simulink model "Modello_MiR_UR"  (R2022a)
settings: Solver=FixedStepAuto  StartTime=0.0  StopTime=time_s(end,1)  FixedStep=Sim.dt*10  RelTol=1e-3  EnableMultiTasking=on
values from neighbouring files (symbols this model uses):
  a = 0.250    (= 0.25)    [Modello_MiR_UR_script.m]    (also in Modello_MiR_2ruote_script.m; Modello_MiR_6ruote_script.m; Modello_MiR_6ruote_validato_script.m)
  a1 = 0.18265    [Modello_MiR_UR_script.m]    (also in UR_DHtable_e.m = 0; Modello_MiR_2ruote_script.m = deg2rad(5); Modello_MiR_6ruote_script.m = deg2rad(5); Modello_MiR_6ruote_validato_script.m)
  a2 = 0.40857    [Modello_MiR_UR_script.m]    (also in UR_DHtable_e.m = 612; Modello_MiR_2ruote_script.m = deg2rad(25); Modello_MiR_6ruote_script.m = deg2rad(25); Modello_MiR_6ruote_validato_script.m)
  Att_C1 = 0.01    [Modello_MiR_UR_script.m]    (also in Modello_MiR_6ruote_validato_script.m)
  Att_C2 = 0.01    [Modello_MiR_UR_script.m]    (also in Modello_MiR_6ruote_validato_script.m)
  Att_C5 = 0.01    [Modello_MiR_UR_script.m]    (also in Modello_MiR_6ruote_validato_script.m)
  Att_C6 = 0.01    [Modello_MiR_UR_script.m]    (also in Modello_MiR_6ruote_validato_script.m)
  b = 0.1875    [Modello_MiR_UR_script.m]    (also in Modello_MiR_2ruote_script.m; Modello_MiR_6ruote_script.m; Modello_MiR_6ruote_validato_script.m)
  b_caster = 0.07    [Modello_MiR_UR_script.m]    (also in Modello_MiR_2ruote_script.m; Modello_MiR_6ruote_script.m; Modello_MiR_6ruote_validato_script.m)
  bd = 0.205    [Modello_MiR_UR_script.m]    (also in Modello_MiR_2ruote_script.m; Modello_MiR_6ruote_script.m; Modello_MiR_6ruote_validato_script.m)
  F23MIR = @(u) (mv*9.801/4)-(mv*h*u(5)+(mv*9.801/4)*(2*a-b_caster*(cos(u(1))+cos(u(2)))))/(4*a-b_caster*(cos(u(1))+cos(u(2)))+b_caster*(cos(u(3))+cos(u(4))))    [Modello_MiR_UR_script.m]
  F23UR5 = @(u) (u(7)/4)-u(11)    [Modello_MiR_UR_script.m]
  F43MIR = @(u) (1/(2*bd))*(mv*u(6)*h+((mv*h*u(5)+(mv*9.801/4)*(2*a-b_caster*(cos(u(1))+cos(u(2)))))/(4*a-b_caster*(cos(u(1))+cos(u(2)))+b_caster*(cos(u(3))+cos(u(4)))))*(2*bd-b_caster*(sin(u(3))+sin(u(4))))+((mv*9.801/4)-(mv*h*u(5)+(mv*9.801/4)*(2*a-b_caster*(cos(u(1))+cos(u(2)))))/(4*a-b_caster*(cos(u(1))+cos(u(2)))+b_caster*(cos(u(3))+cos(u(4)))))*(2*bd-b_caster*(sin(u(1))+sin(u(2)))))    [Modello_MiR_UR_script.m]
  F43UR5 = @(u) (1/(2*bd))*(u(8) - u(6)*H +u(11)*(2*bd-b_caster*(sin(u(3))+sin(u(4))))+u(12)*(2*bd-b_caster*(sin(u(1))+sin(u(2)))))    [Modello_MiR_UR_script.m]
  F63MIR = @(u) (mv*h*u(5)+(mv*9.801/4)*(2*a-b_caster*(cos(u(1))+cos(u(2)))))/(4*a-b_caster*(cos(u(1))+cos(u(2)))+b_caster*(cos(u(3))+cos(u(4))))    [Modello_MiR_UR_script.m]
  F63UR5 = @(u)(-a*u(7)/2 -u(5)*H -u(9) +(u(7)/4)*(2*a-b_caster*(cos(u(1))+cos(u(2)))))/(4*a-b_caster*(cos(u(1))+cos(u(2)))+b_caster*(cos(u(3))+cos(u(4))))    [Modello_MiR_UR_script.m]
  f_c = 0.29564    [Modello_MiR_UR_script.m]    (also in Modello_MiR_6ruote_validato_script.m)
  f_d3 = 0.35846    [Modello_MiR_UR_script.m]    (also in Modello_MiR_6ruote_validato_script.m)
  f_d4 = 0.2333    [Modello_MiR_UR_script.m]    (also in Modello_MiR_6ruote_validato_script.m)
  fa_c = 0.27474    [Modello_MiR_UR_script.m]    (also in Modello_MiR_6ruote_validato_script.m)
  fa_d3 = 0.3694    [Modello_MiR_UR_script.m]    (also in Modello_MiR_6ruote_validato_script.m)
  fa_d4 = 0.28065    [Modello_MiR_UR_script.m]    (also in Modello_MiR_6ruote_validato_script.m)
  fm_fun = @(u) (u <= -am2 || u >= am2) * 0 + (u > -am2 && u <= -am1) * (- u* Mza/(am2 -am1) - Mza* am2/(am2 -am1)) +           + (u > -am1 && u <= am1) * (Mza * u / am1) + (u > am1 && u < am2) * (Mza * u /(am1 -am2) - Mza * am2 /(am1 - am2))    [Modello_MiR_UR_script.m]    (also in Modello_MiR_6ruote_script.m = @(u) (u <= -am2 | u >= am2)*0 + (u > -am2 && u <= -am1)*(- u; Modello_MiR_6ruote_validato_script.m)
  Hi = 1    [UR5e_data.m]
  Icw_1 = 1/2 * mcw * rc^2    (= 0.002004225735)    [Modello_MiR_UR_script.m]    (also in Modello_MiR_2ruote_script.m; Modello_MiR_6ruote_script.m; Modello_MiR_6ruote_validato_script.m)
  Icw_2 = 1/12 * mcw * ec^2 + 1/4 * mcw * rc^2    (= 0.00104098243873)    [Modello_MiR_UR_script.m]    (also in Modello_MiR_2ruote_script.m; Modello_MiR_6ruote_script.m; Modello_MiR_6ruote_validato_script.m)
  Idw_1 = 1/2 * mdw * rd^2    (= 0.00551836278784)    [Modello_MiR_UR_script.m]    (also in Modello_MiR_2ruote_script.m; Transfer_Function_Gol_Gcl.m = Inertia_vect(jj,1); Modello_MiR_6ruote_script.m; Modello_MiR_6ruote_validato_script.m)
  iMax = 20.7*1.1    (= 22.77)    [Modello_MiR_UR_script.m]    (also in Modello_MiR_2ruote_script.m; Modello_MiR_6ruote_script.m; Modello_MiR_6ruote_validato_script.m)
  Iv = mv * (l^2 + w^2)  / 12    (= 6.75343333333)    [Modello_MiR_UR_script.m]    (also in Modello_MiR_2ruote_script.m; Modello_MiR_6ruote_script.m; Modello_MiR_6ruote_validato_script.m = 8.95033333333)
  Kc = 0.15    [Modello_MiR_UR_script.m]    (also in Modello_MiR_2ruote_script.m; Modello_MiR_6ruote_script.m; Modello_MiR_6ruote_validato_script.m)
  Ki_i = 1    [Modello_MiR_UR_script.m]    (also in Modello_MiR_2ruote_script.m; Modello_MiR_6ruote_script.m; Modello_MiR_6ruote_validato_script.m)
  Ki_v = 1    [Modello_MiR_UR_script.m]    (also in Modello_MiR_2ruote_script.m; Modello_MiR_6ruote_script.m; Modello_MiR_6ruote_validato_script.m)
  kk = 0.00005    (= 5e-05)    [Modello_MiR_UR_script.m]    (also in Modello_MiR_2ruote_script.m; Modello_MiR_6ruote_script.m; Modello_MiR_6ruote_validato_script.m)
  Kp_i = 5    [Modello_MiR_UR_script.m]    (also in Modello_MiR_2ruote_script.m; Modello_MiR_6ruote_script.m; Modello_MiR_6ruote_validato_script.m)
  Kp_v = 5    [Modello_MiR_UR_script.m]    (also in Modello_MiR_2ruote_script.m; Modello_MiR_6ruote_script.m; Modello_MiR_6ruote_validato_script.m)
  kv = 1.5e-6    (= 1.5e-06)    [Modello_MiR_UR_script.m]    (also in Modello_MiR_2ruote_script.m; Modello_MiR_6ruote_script.m; Modello_MiR_6ruote_validato_script.m)
  L = R * tauE    (= 0.00181134822805)    [Modello_MiR_UR_script.m]    (also in Modello_MiR_2ruote_script.m; Modello_MiR_6ruote_script.m; Modello_MiR_6ruote_validato_script.m)
  mcw = rc^2 * pi * ec * rhopoliu + 1    (= 1.02616357632)    [Modello_MiR_UR_script.m]    (also in Modello_MiR_2ruote_script.m; Modello_MiR_6ruote_script.m; Modello_MiR_6ruote_validato_script.m)
  mv = 83    [Modello_MiR_UR_script.m]    (also in Modello_MiR_2ruote_script.m; Modello_MiR_6ruote_script.m; Modello_MiR_6ruote_validato_script.m = 110)
  Phi1_start = psi_mir(1,1)    [Modello_MiR_UR_script.m]    (also in Modello_MiR_6ruote_validato_script.m)
  Phi2_start = psi_mir(1,1)    [Modello_MiR_UR_script.m]    (also in Modello_MiR_6ruote_validato_script.m)
  Phi5_start = psi_mir(1,1)    [Modello_MiR_UR_script.m]    (also in Modello_MiR_6ruote_validato_script.m)
  Phi6_start = psi_mir(1,1)    [Modello_MiR_UR_script.m]    (also in Modello_MiR_6ruote_validato_script.m)
  Psi_start = psi_mir(1,1)    [Modello_MiR_UR_script.m]    (also in Modello_MiR_6ruote_script.m = 1.57079632679; Modello_MiR_6ruote_validato_script.m)
  q0 = [qset.q1.signals.values(1),qset.q2.signals.values(1),qset.q3.signals.values(1),qset.q4.signals.values(1),qset.q5.signals.values(1),qset.q6.signals.values(1)]    [UR5e_simmot.m]
  R = velMax * TorqueMax / (iMax)^2    (= 1.81134822805)    [Modello_MiR_UR_script.m]    (also in Modello_MiR_2ruote_script.m; Modello_MiR_6ruote_script.m; Modello_MiR_6ruote_validato_script.m)
  rap_rid = 10.167    [Modello_MiR_UR_script.m]    (also in Modello_MiR_2ruote_script.m; Modello_MiR_6ruote_script.m; Modello_MiR_6ruote_validato_script.m)
  rc = 0.125/2    (= 0.0625)    [Modello_MiR_UR_script.m]    (also in Modello_MiR_2ruote_script.m; Modello_MiR_6ruote_script.m; Modello_MiR_6ruote_validato_script.m)
  rd = 0.1    [Modello_MiR_UR_script.m]    (also in Modello_MiR_2ruote_script.m; Modello_MiR_6ruote_script.m; Modello_MiR_6ruote_validato_script.m)
  s = 1i*s    [Transfer_Function_Gol_Gcl.m]
  s1 = 0.18987    [Modello_MiR_UR_script.m]    (also in Modello_MiR_2ruote_script.m = 0.2; Modello_MiR_6ruote_script.m = 0.2; Modello_MiR_6ruote_validato_script.m)
  s2 = 0.99533    [Modello_MiR_UR_script.m]    (also in Modello_MiR_2ruote_script.m = 0.8; Modello_MiR_6ruote_script.m = 0.8; Modello_MiR_6ruote_validato_script.m)
  Sx = spline(x ,fl_fun(x),zx)    [Modello_MiR_6ruote_script.m]
  Sy = spline(x ,ft_fun(x),zy)    [Modello_MiR_6ruote_script.m]
  tau_i = 1/(2000*2*pi)    (= 7.95774715459e-05)    [UR5e_data.m]    (also in Transfer_Function_Gol_Gcl.m = Kp_i/Ki_i)
  VaMax = Kc * velMax    (= 41.2443991527)    [Modello_MiR_UR_script.m]    (also in Modello_MiR_2ruote_script.m; Modello_MiR_6ruote_script.m; Modello_MiR_6ruote_validato_script.m)
  X_start = traj(1,1)    [Modello_MiR_UR_script.m]    (also in Modello_MiR_2ruote_script.m = input('Inserire coordinata x iniziale'); Modello_MiR_6ruote_script.m = input('Inserire coordinata x iniziale'); Modello_MiR_6ruote_validato_script.m)
  Y_start = traj(1,2)    [Modello_MiR_UR_script.m]    (also in Modello_MiR_2ruote_script.m = input('Inserire coordinata y iniziale'); Modello_MiR_6ruote_script.m = input('Inserire coordinata y iniziale'); Modello_MiR_6ruote_validato_script.m)
undefined symbols (not defined in the file or in its folder): deg, Driver1, Driver2, Driver3, Driver4, Driver5, Driver6, Ground, J1, J2, J3, J4, J5, J6, kg, L1, L2, L3, L4, L5, L6, m, Motor, N, X, Y, z, Z
libraries: sm_lib x33, nesl_utility x30, slpidlib x10
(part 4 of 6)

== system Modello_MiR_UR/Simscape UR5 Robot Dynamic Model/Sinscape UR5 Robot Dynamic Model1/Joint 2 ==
  T2 : Inport
  A_12*E_1 : sm_lib/Frames and Transforms/Rigid Transform  TranslationMethod=Cartesian  TranslationStandardOffset=0  TranslationLengthUnit=mm  TranslationStandardAxis=+Z  TranslationCartesianOffset=A12t  TranslationROffset=0  TranslationROffsetUnits=m  TranslationZOffset=0  TranslationZOffsetUnits=m  TranslationThetaOffset=0  TranslationThetaOffsetUnits=deg  RotationMethod=None  RotationAngleUnits=deg  RotationStandardAxis=+Z  RotationAngle=0.0  RotationArbitraryAxis=[0 0 1]  FollAlignAxisA=+X  BaseAlignAxisA=+Y  FollAlignAxisB=+Y  BaseAlignAxisB=+Z  RotationSequenceAxes=FollowerAxes  RotationSequence=XYX  RotationSequenceAngles=[0 0 0]  RotationSequenceAnglesUnits=deg  RotationMatrix=A12r
  A_12*E_12 : sm_lib/Frames and Transforms/Rigid Transform  TranslationMethod=None  TranslationStandardOffset=0  TranslationLengthUnit=mm  TranslationStandardAxis=+Z  TranslationCartesianOffset=A12t  TranslationROffset=0  TranslationROffsetUnits=m  TranslationZOffset=0  TranslationZOffsetUnits=m  TranslationThetaOffset=0  TranslationThetaOffsetUnits=deg  RotationMethod=RotationMatrix  RotationAngleUnits=deg  RotationStandardAxis=+Z  RotationAngle=0.0  RotationArbitraryAxis=[0 0 1]  FollAlignAxisA=+X  BaseAlignAxisA=+Y  FollAlignAxisB=+Y  BaseAlignAxisB=+Z  RotationSequenceAxes=FollowerAxes  RotationSequence=XYX  RotationSequenceAngles=[0 0 0]  RotationSequenceAnglesUnits=deg  RotationMatrix=A12r
  Mux : Mux  Inputs=3
  PS-Simulink Converter1 : nesl_utility/PS-Simulink Converter  PhysicalDomain=network_engine_domain  SubClassName=ps_output  LeftPortType=input  RightPortType=output  PseudoPeriodic=off  Frequencies=[]  VectorFormat=1-D array  Unit=1  AffineConversion=off
  PS-Simulink Converter2 : nesl_utility/PS-Simulink Converter  PhysicalDomain=network_engine_domain  SubClassName=ps_output  LeftPortType=input  RightPortType=output  PseudoPeriodic=off  Frequencies=[]  VectorFormat=1-D array  Unit=1  AffineConversion=off
  PS-Simulink Converter7 : nesl_utility/PS-Simulink Converter  PhysicalDomain=network_engine_domain  SubClassName=ps_output  LeftPortType=input  RightPortType=output  PseudoPeriodic=off  Frequencies=[]  VectorFormat=1-D array  Unit=1  AffineConversion=off
  Revolute Joint2 : sm_lib/Joints/Revolute Joint  JointMode=Normal  SenseConstraintForce=off  SenseConstraintForceX=off  SenseConstraintForceY=off  SenseConstraintForceZ=off  SenseConstraintTorque=off  SenseConstraintTorqueX=off  SenseConstraintTorqueY=off  SenseConstraintTorqueZ=off  SenseTotalForce=off  SenseTotalForceX=off  SenseTotalForceY=off  SenseTotalForceZ=off  SenseTotalTorque=off  SenseTotalTorqueX=off  SenseTotalTorqueY=off  SenseTotalTorqueZ=off  CompositeWrenchDir=FollowerOnBase  CompositeWrenchFrame=BaseFrame  EquilibriumPosition=0  EquilibriumPositionUnits=deg  SpringStiffness=0  SpringStiffnessUnits=N*m/deg  DampingCoefficient=0  DampingCoefficientUnits=N*m/(deg/s)  TorqueActuationMode=InputTorque  MotionActuationMode=ComputedMotion  SensePosition=on  SenseVelocity=on  SenseAcceleration=on  SenseTorqueForce=off  SenseLowerLimitTorqueForce=off  SenseUpperLimitTorqueForce=off  LowerLimitSpecify=on  LowerLimitBound=-J2.al  LowerLimitBoundUnits=deg  LowerLimitStiffness=1e4  LowerLimitStiffnessUnits=N*m/deg  LowerLimitDamping=10  LowerLimitDampingUnits=N*m/(deg/s)  LowerLimitTransitionRegionWidth=0.1  LowerLimitTransitionRegionWidthUnits=deg  UpperLimitSpecify=on  UpperLimitBound=J2.al  UpperLimitBoundUnits=deg  UpperLimitStiffness=1e4  UpperLimitStiffnessUnits=N*m/deg  UpperLimitDamping=10  UpperLimitDampingUnits=N*m/(deg/s)  UpperLimitTransitionRegionWidth=0.1  UpperLimitTransitionRegionWidthUnits=deg  PositionTargetSpecify=on  PositionTargetPriority=High  PositionTargetValue=q0(2)  PositionTargetValueUnits=rad  VelocityTargetSpecify=off  VelocityTargetPriority=High  VelocityTargetValue=0  VelocityTargetValueUnits=deg/s
  Simulink-PS Converter : nesl_utility/Simulink-PS Converter  PhysicalDomain=network_engine_domain  SubClassName=ps_input  LeftPortType=input  RightPortType=output  PseudoPeriodic=off  Frequencies=[]  NoiseDistribution=none  NoiseParameters=[]  Unit=1  AffineConversion=off  FilteringAndDerivatives=provide  SimscapeFilterOrder=1  InputFilterTimeConstant=0.001  UdotUserProvided=0
  Link 1 : PMIOPort  Side=Left
  Link 2 : PMIOPort  Port=2  Side=Right
  q2,qd2,qdd2 : Outport
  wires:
  PS-Simulink Converter1/1 -> Mux/1
  T2/1 -> Simulink-PS Converter/1
  Mux/1 -> q2,qd2,qdd2/1
  PS-Simulink Converter7/1 -> Mux/2
  PS-Simulink Converter2/1 -> Mux/3
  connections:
  Revolute Joint2/LConn1 -- A_12*E_1/RConn1
  A_12*E_1/LConn1 -- A_12*E_12/RConn1
  Revolute Joint2/RConn1 -- Link 2/RConn1
  A_12*E_12/LConn1 -- Link 1/RConn1
  Revolute Joint2/RConn4 -- PS-Simulink Converter2/LConn1
  Revolute Joint2/LConn2 -- Simulink-PS Converter/RConn1
  Revolute Joint2/RConn3 -- PS-Simulink Converter7/LConn1
  Revolute Joint2/RConn2 -- PS-Simulink Converter1/LConn1

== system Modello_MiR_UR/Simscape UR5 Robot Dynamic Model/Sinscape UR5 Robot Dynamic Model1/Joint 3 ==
  T3 : Inport
  A_23*E_1 : sm_lib/Frames and Transforms/Rigid Transform  TranslationMethod=Cartesian  TranslationStandardOffset=0  TranslationLengthUnit=mm  TranslationStandardAxis=+Z  TranslationCartesianOffset=A23t  TranslationROffset=0  TranslationROffsetUnits=m  TranslationZOffset=0  TranslationZOffsetUnits=m  TranslationThetaOffset=0  TranslationThetaOffsetUnits=deg  RotationMethod=None  RotationAngleUnits=deg  RotationStandardAxis=+Z  RotationAngle=0.0  RotationArbitraryAxis=[0 0 1]  FollAlignAxisA=+X  BaseAlignAxisA=+Y  FollAlignAxisB=+Y  BaseAlignAxisB=+Z  RotationSequenceAxes=FollowerAxes  RotationSequence=XYX  RotationSequenceAngles=[0 0 0]  RotationSequenceAnglesUnits=deg  RotationMatrix=A23r
  A_23*E_23 : sm_lib/Frames and Transforms/Rigid Transform  TranslationMethod=None  TranslationStandardOffset=0  TranslationLengthUnit=mm  TranslationStandardAxis=+Z  TranslationCartesianOffset=A23t  TranslationROffset=0  TranslationROffsetUnits=m  TranslationZOffset=0  TranslationZOffsetUnits=m  TranslationThetaOffset=0  TranslationThetaOffsetUnits=deg  RotationMethod=RotationMatrix  RotationAngleUnits=deg  RotationStandardAxis=+Z  RotationAngle=0.0  RotationArbitraryAxis=[0 0 1]  FollAlignAxisA=+X  BaseAlignAxisA=+Y  FollAlignAxisB=+Y  BaseAlignAxisB=+Z  RotationSequenceAxes=FollowerAxes  RotationSequence=XYX  RotationSequenceAngles=[0 0 0]  RotationSequenceAnglesUnits=deg  RotationMatrix=A23r
  Mux : Mux  Inputs=3
  PS-Simulink Converter1 : nesl_utility/PS-Simulink Converter  PhysicalDomain=network_engine_domain  SubClassName=ps_output  LeftPortType=input  RightPortType=output  PseudoPeriodic=off  Frequencies=[]  VectorFormat=1-D array  Unit=1  AffineConversion=off
  PS-Simulink Converter2 : nesl_utility/PS-Simulink Converter  PhysicalDomain=network_engine_domain  SubClassName=ps_output  LeftPortType=input  RightPortType=output  PseudoPeriodic=off  Frequencies=[]  VectorFormat=1-D array  Unit=1  AffineConversion=off
  PS-Simulink Converter7 : nesl_utility/PS-Simulink Converter  PhysicalDomain=network_engine_domain  SubClassName=ps_output  LeftPortType=input  RightPortType=output  PseudoPeriodic=off  Frequencies=[]  VectorFormat=1-D array  Unit=1  AffineConversion=off
  Revolute Joint3 : sm_lib/Joints/Revolute Joint  JointMode=Normal  SenseConstraintForce=off  SenseConstraintForceX=off  SenseConstraintForceY=off  SenseConstraintForceZ=off  SenseConstraintTorque=off  SenseConstraintTorqueX=off  SenseConstraintTorqueY=off  SenseConstraintTorqueZ=off  SenseTotalForce=off  SenseTotalForceX=off  SenseTotalForceY=off  SenseTotalForceZ=off  SenseTotalTorque=off  SenseTotalTorqueX=off  SenseTotalTorqueY=off  SenseTotalTorqueZ=off  CompositeWrenchDir=FollowerOnBase  CompositeWrenchFrame=BaseFrame  EquilibriumPosition=0  EquilibriumPositionUnits=deg  SpringStiffness=0  SpringStiffnessUnits=N*m/deg  DampingCoefficient=0  DampingCoefficientUnits=N*m/(deg/s)  TorqueActuationMode=InputTorque  MotionActuationMode=ComputedMotion  SensePosition=on  SenseVelocity=on  SenseAcceleration=on  SenseTorqueForce=off  SenseLowerLimitTorqueForce=off  SenseUpperLimitTorqueForce=off  LowerLimitSpecify=on  LowerLimitBound=-J3.al  LowerLimitBoundUnits=deg  LowerLimitStiffness=1e4  LowerLimitStiffnessUnits=N*m/deg  LowerLimitDamping=10  LowerLimitDampingUnits=N*m/(deg/s)  LowerLimitTransitionRegionWidth=0.1  LowerLimitTransitionRegionWidthUnits=deg  UpperLimitSpecify=on  UpperLimitBound=J3.al  UpperLimitBoundUnits=deg  UpperLimitStiffness=1e4  UpperLimitStiffnessUnits=N*m/deg  UpperLimitDamping=10  UpperLimitDampingUnits=N*m/(deg/s)  UpperLimitTransitionRegionWidth=0.1  UpperLimitTransitionRegionWidthUnits=deg  PositionTargetSpecify=on  PositionTargetPriority=High  PositionTargetValue=q0(3)  PositionTargetValueUnits=rad  VelocityTargetSpecify=off  VelocityTargetPriority=High  VelocityTargetValue=0  VelocityTargetValueUnits=deg/s
  Simulink-PS Converter : nesl_utility/Simulink-PS Converter  PhysicalDomain=network_engine_domain  SubClassName=ps_input  LeftPortType=input  RightPortType=output  PseudoPeriodic=off  Frequencies=[]  NoiseDistribution=none  NoiseParameters=[]  Unit=1  AffineConversion=off  FilteringAndDerivatives=provide  SimscapeFilterOrder=1  InputFilterTimeConstant=0.001  UdotUserProvided=0
  Link 2 : PMIOPort  Side=Left
  Link 3 : PMIOPort  Port=2  Side=Right
  q3,qd3,qdd3 : Outport
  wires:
  PS-Simulink Converter1/1 -> Mux/1
  T3/1 -> Simulink-PS Converter/1
  Mux/1 -> q3,qd3,qdd3/1
  PS-Simulink Converter7/1 -> Mux/2
  PS-Simulink Converter2/1 -> Mux/3
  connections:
  A_23*E_1/RConn1 -- Revolute Joint3/LConn1
  A_23*E_1/LConn1 -- A_23*E_23/RConn1
  A_23*E_23/LConn1 -- Link 2/RConn1
  Revolute Joint3/RConn1 -- Link 3/RConn1
  Revolute Joint3/RConn4 -- PS-Simulink Converter2/LConn1
  Revolute Joint3/LConn2 -- Simulink-PS Converter/RConn1
  Revolute Joint3/RConn3 -- PS-Simulink Converter7/LConn1
  Revolute Joint3/RConn2 -- PS-Simulink Converter1/LConn1

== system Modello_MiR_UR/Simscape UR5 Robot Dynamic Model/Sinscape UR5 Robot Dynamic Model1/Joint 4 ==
  T4 : Inport
  A_34*E_1 : sm_lib/Frames and Transforms/Rigid Transform  TranslationMethod=Cartesian  TranslationStandardOffset=0  TranslationLengthUnit=mm  TranslationStandardAxis=+Z  TranslationCartesianOffset=A34t  TranslationROffset=0  TranslationROffsetUnits=m  TranslationZOffset=0  TranslationZOffsetUnits=m  TranslationThetaOffset=0  TranslationThetaOffsetUnits=deg  RotationMethod=None  RotationAngleUnits=deg  RotationStandardAxis=+Z  RotationAngle=0.0  RotationArbitraryAxis=[0 0 1]  FollAlignAxisA=+X  BaseAlignAxisA=+Y  FollAlignAxisB=+Y  BaseAlignAxisB=+Z  RotationSequenceAxes=FollowerAxes  RotationSequence=XYX  RotationSequenceAngles=[0 0 0]  RotationSequenceAnglesUnits=deg  RotationMatrix=A34r
  A_34*E_34 : sm_lib/Frames and Transforms/Rigid Transform  TranslationMethod=None  TranslationStandardOffset=0  TranslationLengthUnit=mm  TranslationStandardAxis=+Z  TranslationCartesianOffset=A34t  TranslationROffset=0  TranslationROffsetUnits=m  TranslationZOffset=0  TranslationZOffsetUnits=m  TranslationThetaOffset=0  TranslationThetaOffsetUnits=deg  RotationMethod=RotationMatrix  RotationAngleUnits=deg  RotationStandardAxis=+Z  RotationAngle=0.0  RotationArbitraryAxis=[0 0 1]  FollAlignAxisA=+X  BaseAlignAxisA=+Y  FollAlignAxisB=+Y  BaseAlignAxisB=+Z  RotationSequenceAxes=FollowerAxes  RotationSequence=XYX  RotationSequenceAngles=[0 0 0]  RotationSequenceAnglesUnits=deg  RotationMatrix=A34r
  Mux : Mux  Inputs=3
  PS-Simulink Converter1 : nesl_utility/PS-Simulink Converter  PhysicalDomain=network_engine_domain  SubClassName=ps_output  LeftPortType=input  RightPortType=output  PseudoPeriodic=off  Frequencies=[]  VectorFormat=1-D array  Unit=1  AffineConversion=off
  PS-Simulink Converter2 : nesl_utility/PS-Simulink Converter  PhysicalDomain=network_engine_domain  SubClassName=ps_output  LeftPortType=input  RightPortType=output  PseudoPeriodic=off  Frequencies=[]  VectorFormat=1-D array  Unit=1  AffineConversion=off
  PS-Simulink Converter7 : nesl_utility/PS-Simulink Converter  PhysicalDomain=network_engine_domain  SubClassName=ps_output  LeftPortType=input  RightPortType=output  PseudoPeriodic=off  Frequencies=[]  VectorFormat=1-D array  Unit=1  AffineConversion=off
  Revolute Joint4 : sm_lib/Joints/Revolute Joint  JointMode=Normal  SenseConstraintForce=off  SenseConstraintForceX=off  SenseConstraintForceY=off  SenseConstraintForceZ=off  SenseConstraintTorque=off  SenseConstraintTorqueX=off  SenseConstraintTorqueY=off  SenseConstraintTorqueZ=off  SenseTotalForce=off  SenseTotalForceX=off  SenseTotalForceY=off  SenseTotalForceZ=off  SenseTotalTorque=off  SenseTotalTorqueX=off  SenseTotalTorqueY=off  SenseTotalTorqueZ=off  CompositeWrenchDir=FollowerOnBase  CompositeWrenchFrame=BaseFrame  EquilibriumPosition=0  EquilibriumPositionUnits=deg  SpringStiffness=0  SpringStiffnessUnits=N*m/deg  DampingCoefficient=0  DampingCoefficientUnits=N*m/(deg/s)  TorqueActuationMode=InputTorque  MotionActuationMode=ComputedMotion  SensePosition=on  SenseVelocity=on  SenseAcceleration=on  SenseTorqueForce=off  SenseLowerLimitTorqueForce=off  SenseUpperLimitTorqueForce=off  LowerLimitSpecify=on  LowerLimitBound=-J4.al  LowerLimitBoundUnits=deg  LowerLimitStiffness=1e4  LowerLimitStiffnessUnits=N*m/deg  LowerLimitDamping=10  LowerLimitDampingUnits=N*m/(deg/s)  LowerLimitTransitionRegionWidth=0.1  LowerLimitTransitionRegionWidthUnits=deg  UpperLimitSpecify=on  UpperLimitBound=J4.al  UpperLimitBoundUnits=deg  UpperLimitStiffness=1e4  UpperLimitStiffnessUnits=N*m/deg  UpperLimitDamping=10  UpperLimitDampingUnits=N*m/(deg/s)  UpperLimitTransitionRegionWidth=0.1  UpperLimitTransitionRegionWidthUnits=deg  PositionTargetSpecify=on  PositionTargetPriority=High  PositionTargetValue=q0(4)  PositionTargetValueUnits=rad  VelocityTargetSpecify=off  VelocityTargetPriority=High  VelocityTargetValue=0  VelocityTargetValueUnits=deg/s
  Simulink-PS Converter : nesl_utility/Simulink-PS Converter  PhysicalDomain=network_engine_domain  SubClassName=ps_input  LeftPortType=input  RightPortType=output  PseudoPeriodic=off  Frequencies=[]  NoiseDistribution=none  NoiseParameters=[]  Unit=1  AffineConversion=off  FilteringAndDerivatives=provide  SimscapeFilterOrder=1  InputFilterTimeConstant=0.001  UdotUserProvided=0
  Link 3 : PMIOPort  Side=Left
  Link 4 : PMIOPort  Port=2  Side=Right
  q4,qd4,qdd4 : Outport
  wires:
  PS-Simulink Converter1/1 -> Mux/1
  T4/1 -> Simulink-PS Converter/1
  Mux/1 -> q4,qd4,qdd4/1
  PS-Simulink Converter7/1 -> Mux/2
  PS-Simulink Converter2/1 -> Mux/3
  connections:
  A_34*E_1/LConn1 -- A_34*E_34/RConn1
  A_34*E_1/RConn1 -- Revolute Joint4/LConn1
  Link 3/RConn1 -- A_34*E_34/LConn1
  Revolute Joint4/RConn1 -- Link 4/RConn1
  Revolute Joint4/RConn4 -- PS-Simulink Converter2/LConn1
  Revolute Joint4/LConn2 -- Simulink-PS Converter/RConn1
  Revolute Joint4/RConn3 -- PS-Simulink Converter7/LConn1
  Revolute Joint4/RConn2 -- PS-Simulink Converter1/LConn1

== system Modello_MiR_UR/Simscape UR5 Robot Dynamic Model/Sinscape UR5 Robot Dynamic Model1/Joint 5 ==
  T5 : Inport
  A_45*E_1 : sm_lib/Frames and Transforms/Rigid Transform  TranslationMethod=Cartesian  TranslationStandardOffset=0  TranslationLengthUnit=mm  TranslationStandardAxis=+Z  TranslationCartesianOffset=A45t  TranslationROffset=0  TranslationROffsetUnits=m  TranslationZOffset=0  TranslationZOffsetUnits=m  TranslationThetaOffset=0  TranslationThetaOffsetUnits=deg  RotationMethod=None  RotationAngleUnits=deg  RotationStandardAxis=+Z  RotationAngle=0.0  RotationArbitraryAxis=[0 0 1]  FollAlignAxisA=+X  BaseAlignAxisA=+Y  FollAlignAxisB=+Y  BaseAlignAxisB=+Z  RotationSequenceAxes=FollowerAxes  RotationSequence=XYX  RotationSequenceAngles=[0 0 0]  RotationSequenceAnglesUnits=deg  RotationMatrix=A45r
  A_45*E_45 : sm_lib/Frames and Transforms/Rigid Transform  TranslationMethod=None  TranslationStandardOffset=0  TranslationLengthUnit=mm  TranslationStandardAxis=+Z  TranslationCartesianOffset=A45t  TranslationROffset=0  TranslationROffsetUnits=m  TranslationZOffset=0  TranslationZOffsetUnits=m  TranslationThetaOffset=0  TranslationThetaOffsetUnits=deg  RotationMethod=RotationMatrix  RotationAngleUnits=deg  RotationStandardAxis=+Z  RotationAngle=0.0  RotationArbitraryAxis=[0 0 1]  FollAlignAxisA=+X  BaseAlignAxisA=+Y  FollAlignAxisB=+Y  BaseAlignAxisB=+Z  RotationSequenceAxes=FollowerAxes  RotationSequence=XYX  RotationSequenceAngles=[0 0 0]  RotationSequenceAnglesUnits=deg  RotationMatrix=A45r
  Mux : Mux  Inputs=3
  PS-Simulink Converter1 : nesl_utility/PS-Simulink Converter  PhysicalDomain=network_engine_domain  SubClassName=ps_output  LeftPortType=input  RightPortType=output  PseudoPeriodic=off  Frequencies=[]  VectorFormat=1-D array  Unit=1  AffineConversion=off
  PS-Simulink Converter2 : nesl_utility/PS-Simulink Converter  PhysicalDomain=network_engine_domain  SubClassName=ps_output  LeftPortType=input  RightPortType=output  PseudoPeriodic=off  Frequencies=[]  VectorFormat=1-D array  Unit=1  AffineConversion=off
  PS-Simulink Converter7 : nesl_utility/PS-Simulink Converter  PhysicalDomain=network_engine_domain  SubClassName=ps_output  LeftPortType=input  RightPortType=output  PseudoPeriodic=off  Frequencies=[]  VectorFormat=1-D array  Unit=1  AffineConversion=off
  Revolute Joint5 : sm_lib/Joints/Revolute Joint  JointMode=Normal  SenseConstraintForce=off  SenseConstraintForceX=off  SenseConstraintForceY=off  SenseConstraintForceZ=off  SenseConstraintTorque=off  SenseConstraintTorqueX=off  SenseConstraintTorqueY=off  SenseConstraintTorqueZ=off  SenseTotalForce=off  SenseTotalForceX=off  SenseTotalForceY=off  SenseTotalForceZ=off  SenseTotalTorque=off  SenseTotalTorqueX=off  SenseTotalTorqueY=off  SenseTotalTorqueZ=off  CompositeWrenchDir=FollowerOnBase  CompositeWrenchFrame=BaseFrame  EquilibriumPosition=0  EquilibriumPositionUnits=deg  SpringStiffness=0  SpringStiffnessUnits=N*m/deg  DampingCoefficient=0  DampingCoefficientUnits=N*m/(deg/s)  TorqueActuationMode=InputTorque  MotionActuationMode=ComputedMotion  SensePosition=on  SenseVelocity=on  SenseAcceleration=on  SenseTorqueForce=off  SenseLowerLimitTorqueForce=off  SenseUpperLimitTorqueForce=off  LowerLimitSpecify=on  LowerLimitBound=-J5.al  LowerLimitBoundUnits=deg  LowerLimitStiffness=1e4  LowerLimitStiffnessUnits=N*m/deg  LowerLimitDamping=10  LowerLimitDampingUnits=N*m/(deg/s)  LowerLimitTransitionRegionWidth=0.1  LowerLimitTransitionRegionWidthUnits=deg  UpperLimitSpecify=on  UpperLimitBound=J5.al  UpperLimitBoundUnits=deg  UpperLimitStiffness=1e4  UpperLimitStiffnessUnits=N*m/deg  UpperLimitDamping=10  UpperLimitDampingUnits=N*m/(deg/s)  UpperLimitTransitionRegionWidth=0.1  UpperLimitTransitionRegionWidthUnits=deg  PositionTargetSpecify=on  PositionTargetPriority=High  PositionTargetValue=q0(5)  PositionTargetValueUnits=rad  VelocityTargetSpecify=off  VelocityTargetPriority=High  VelocityTargetValue=0  VelocityTargetValueUnits=deg/s
  Simulink-PS Converter : nesl_utility/Simulink-PS Converter  PhysicalDomain=network_engine_domain  SubClassName=ps_input  LeftPortType=input  RightPortType=output  PseudoPeriodic=off  Frequencies=[]  NoiseDistribution=none  NoiseParameters=[]  Unit=1  AffineConversion=off  FilteringAndDerivatives=provide  SimscapeFilterOrder=1  InputFilterTimeConstant=0.001  UdotUserProvided=0
  Link 4 : PMIOPort  Side=Left
  Link 5 : PMIOPort  Port=2  Side=Right
  q5,qd5,qdd5 : Outport
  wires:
  PS-Simulink Converter1/1 -> Mux/1
  T5/1 -> Simulink-PS Converter/1
  Mux/1 -> q5,qd5,qdd5/1
  PS-Simulink Converter7/1 -> Mux/2
  PS-Simulink Converter2/1 -> Mux/3
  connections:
  A_45*E_45/RConn1 -- A_45*E_1/LConn1
  A_45*E_1/RConn1 -- Revolute Joint5/LConn1
  A_45*E_45/LConn1 -- Link 4/RConn1
  Revolute Joint5/RConn1 -- Link 5/RConn1
  Revolute Joint5/RConn4 -- PS-Simulink Converter2/LConn1
  Revolute Joint5/LConn2 -- Simulink-PS Converter/RConn1
  Revolute Joint5/RConn3 -- PS-Simulink Converter7/LConn1
  Revolute Joint5/RConn2 -- PS-Simulink Converter1/LConn1

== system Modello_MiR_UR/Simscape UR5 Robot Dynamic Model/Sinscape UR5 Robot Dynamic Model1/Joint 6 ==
  T6 : Inport
  A_56*E_1 : sm_lib/Frames and Transforms/Rigid Transform  TranslationMethod=Cartesian  TranslationStandardOffset=0  TranslationLengthUnit=mm  TranslationStandardAxis=+Z  TranslationCartesianOffset=A56t  TranslationROffset=0  TranslationROffsetUnits=m  TranslationZOffset=0  TranslationZOffsetUnits=m  TranslationThetaOffset=0  TranslationThetaOffsetUnits=deg  RotationMethod=None  RotationAngleUnits=deg  RotationStandardAxis=+Z  RotationAngle=0.0  RotationArbitraryAxis=[0 0 1]  FollAlignAxisA=+X  BaseAlignAxisA=+Y  FollAlignAxisB=+Y  BaseAlignAxisB=+Z  RotationSequenceAxes=FollowerAxes  RotationSequence=XYX  RotationSequenceAngles=[0 0 0]  RotationSequenceAnglesUnits=deg  RotationMatrix=A56r
  A_56*E_56 : sm_lib/Frames and Transforms/Rigid Transform  TranslationMethod=None  TranslationStandardOffset=0  TranslationLengthUnit=mm  TranslationStandardAxis=+Z  TranslationCartesianOffset=A56t  TranslationROffset=0  TranslationROffsetUnits=m  TranslationZOffset=0  TranslationZOffsetUnits=m  TranslationThetaOffset=0  TranslationThetaOffsetUnits=deg  RotationMethod=RotationMatrix  RotationAngleUnits=deg  RotationStandardAxis=+Z  RotationAngle=0.0  RotationArbitraryAxis=[0 0 1]  FollAlignAxisA=+X  BaseAlignAxisA=+Y  FollAlignAxisB=+Y  BaseAlignAxisB=+Z  RotationSequenceAxes=FollowerAxes  RotationSequence=XYX  RotationSequenceAngles=[0 0 0]  RotationSequenceAnglesUnits=deg  RotationMatrix=A56r
  Mux : Mux  Inputs=3
  PS-Simulink Converter1 : nesl_utility/PS-Simulink Converter  PhysicalDomain=network_engine_domain  SubClassName=ps_output  LeftPortType=input  RightPortType=output  PseudoPeriodic=off  Frequencies=[]  VectorFormat=1-D array  Unit=1  AffineConversion=off
  PS-Simulink Converter2 : nesl_utility/PS-Simulink Converter  PhysicalDomain=network_engine_domain  SubClassName=ps_output  LeftPortType=input  RightPortType=output  PseudoPeriodic=off  Frequencies=[]  VectorFormat=1-D array  Unit=1  AffineConversion=off
  PS-Simulink Converter7 : nesl_utility/PS-Simulink Converter  PhysicalDomain=network_engine_domain  SubClassName=ps_output  LeftPortType=input  RightPortType=output  PseudoPeriodic=off  Frequencies=[]  VectorFormat=1-D array  Unit=1  AffineConversion=off
  Revolute Joint6 : sm_lib/Joints/Revolute Joint  JointMode=Normal  SenseConstraintForce=off  SenseConstraintForceX=off  SenseConstraintForceY=off  SenseConstraintForceZ=off  SenseConstraintTorque=off  SenseConstraintTorqueX=off  SenseConstraintTorqueY=off  SenseConstraintTorqueZ=off  SenseTotalForce=off  SenseTotalForceX=off  SenseTotalForceY=off  SenseTotalForceZ=off  SenseTotalTorque=off  SenseTotalTorqueX=off  SenseTotalTorqueY=off  SenseTotalTorqueZ=off  CompositeWrenchDir=FollowerOnBase  CompositeWrenchFrame=BaseFrame  EquilibriumPosition=0  EquilibriumPositionUnits=deg  SpringStiffness=0  SpringStiffnessUnits=N*m/deg  DampingCoefficient=0  DampingCoefficientUnits=N*m/(deg/s)  TorqueActuationMode=InputTorque  MotionActuationMode=ComputedMotion  SensePosition=on  SenseVelocity=on  SenseAcceleration=on  SenseTorqueForce=off  SenseLowerLimitTorqueForce=off  SenseUpperLimitTorqueForce=off  LowerLimitSpecify=on  LowerLimitBound=-J6.al  LowerLimitBoundUnits=deg  LowerLimitStiffness=1e4  LowerLimitStiffnessUnits=N*m/deg  LowerLimitDamping=10  LowerLimitDampingUnits=N*m/(deg/s)  LowerLimitTransitionRegionWidth=0.1  LowerLimitTransitionRegionWidthUnits=deg  UpperLimitSpecify=on  UpperLimitBound=J6.al  UpperLimitBoundUnits=deg  UpperLimitStiffness=1e4  UpperLimitStiffnessUnits=N*m/deg  UpperLimitDamping=10  UpperLimitDampingUnits=N*m/(deg/s)  UpperLimitTransitionRegionWidth=0.1  UpperLimitTransitionRegionWidthUnits=deg  PositionTargetSpecify=on  PositionTargetPriority=High  PositionTargetValue=q0(6)  PositionTargetValueUnits=rad  VelocityTargetSpecify=off  VelocityTargetPriority=High  VelocityTargetValue=0  VelocityTargetValueUnits=deg/s
  Simulink-PS Converter : nesl_utility/Simulink-PS Converter  PhysicalDomain=network_engine_domain  SubClassName=ps_input  LeftPortType=input  RightPortType=output  PseudoPeriodic=off  Frequencies=[]  NoiseDistribution=none  NoiseParameters=[]  Unit=1  AffineConversion=off  FilteringAndDerivatives=provide  SimscapeFilterOrder=1  InputFilterTimeConstant=0.001  UdotUserProvided=0
  Link 5 : PMIOPort  Side=Left
  Link 6 : PMIOPort  Port=2  Side=Right
  q6,qd6,qdd6 : Outport
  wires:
  PS-Simulink Converter1/1 -> Mux/1
  T6/1 -> Simulink-PS Converter/1
  Mux/1 -> q6,qd6,qdd6/1
  PS-Simulink Converter7/1 -> Mux/2
  PS-Simulink Converter2/1 -> Mux/3
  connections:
  A_56*E_1/LConn1 -- A_56*E_56/RConn1
  Revolute Joint6/LConn1 -- A_56*E_1/RConn1
  Revolute Joint6/RConn1 -- Link 6/RConn1
  A_56*E_56/LConn1 -- Link 5/RConn1
  Revolute Joint6/RConn4 -- PS-Simulink Converter2/LConn1
  Revolute Joint6/LConn2 -- Simulink-PS Converter/RConn1
  Revolute Joint6/RConn3 -- PS-Simulink Converter7/LConn1
  Revolute Joint6/RConn2 -- PS-Simulink Converter1/LConn1

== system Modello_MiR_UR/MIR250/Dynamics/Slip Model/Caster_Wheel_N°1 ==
  Thetad_1 : Inport
  vx_ruota1 : Inport  Port=2
  gamma1 : Inport  Port=3
  Delta1 : Inport  Port=4
  Confronto velocità ruota 1 : Scope
  Cos : Trigonometry  Operator=cos
  Gain : Gain  Gain=rc
  MATLAB Function1 : MATLAB Function  TreatAsAtomicUnit=on
  MATLAB Function4 : MATLAB Function  TreatAsAtomicUnit=on
  Mux : Mux  Inputs=2
  Product : Product
  Saturation : Saturate  UpperLimit=1  LowerLimit=-1
  Saturation1 : Saturate  UpperLimit=1  LowerLimit=-1
  Scope{,1..5} (6 alike) : Scope
  Sum : Sum  Inputs=|+-
  Switch : Switch
  Sigma1 : Outport
  alpha1 : Outport  Port=2
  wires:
  Thetad_1/1 -> Gain/1
  Gain/1 -> Mux/1, MATLAB Function4/1(v_wheel), MATLAB Function1/1(v_wheel)  "V_wheel"
  Switch/1 -> Scope/1, Sigma1/1
  MATLAB Function1/1(Fc_pos_out) -> Saturation/1
  MATLAB Function4/1(Fc_neg_out) -> Saturation1/1, Scope3/1
  vx_ruota1/1 -> Product/1, Mux/2  "xd_ruota1"
  Delta1/1 -> Sum/2
  Sum/1 -> Cos/1, Scope1/1, alpha1/1, Scope5/1  "alpha1"
  Mux/1 -> Confronto velocità ruota 1/1
  Saturation/1 -> Scope2/1, Switch/1, Switch/2
  Saturation1/1 -> Switch/3
  gamma1/1 -> Scope4/1, Sum/1
  Product/1 -> MATLAB Function1/2(Vx_DL), MATLAB Function4/2(Vx_DL)
  Cos/1 -> Product/2

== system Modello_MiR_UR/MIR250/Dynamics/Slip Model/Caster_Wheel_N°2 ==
  Thetad_2 : Inport
  vx_ruota2 : Inport  Port=2
  gamma2 : Inport  Port=3
  Delta2 : Inport  Port=4
  Cos : Trigonometry  Operator=cos
  Gain : Gain  Gain=rc
  MATLAB Function1 : MATLAB Function  TreatAsAtomicUnit=on
  MATLAB Function2 : MATLAB Function  TreatAsAtomicUnit=on
  Product : Product
  Saturation : Saturate  UpperLimit=1  LowerLimit=-1
  Saturation1 : Saturate  UpperLimit=1  LowerLimit=-1
  Scope{,1..5} (6 alike) : Scope
  Sum : Sum  Inputs=|+-
  Switch : Switch
  Sigma2 : Outport
  alpha2 : Outport  Port=2
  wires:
  Thetad_2/1 -> Gain/1
  gamma2/1 -> Scope4/1, Sum/1
  Gain/1 -> MATLAB Function2/1(v_wheel), MATLAB Function1/1(v_wheel)  "V_wheel"
  Switch/1 -> Scope/1, Sigma2/1
  MATLAB Function1/1(Fc_pos_out) -> Saturation1/1
  MATLAB Function2/1(Fc_neg_out) -> Saturation/1, Scope3/1
  Delta2/1 -> Sum/2
  Saturation1/1 -> Scope2/1, Switch/2, Switch/1
  Saturation/1 -> Switch/3
  Cos/1 -> Product/2
  Sum/1 -> Cos/1, Scope1/1, alpha2/1, Scope5/1  "alpha1"
  Product/1 -> MATLAB Function1/2(Vx_DL), MATLAB Function2/2(Vx_DL)
  vx_ruota2/1 -> Product/1  "vx_ruota2"

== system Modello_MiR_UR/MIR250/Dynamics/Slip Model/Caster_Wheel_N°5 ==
  Thetad_5 : Inport
  vx_ruota5 : Inport  Port=2
  gamma5 : Inport  Port=3
  Delta5 : Inport  Port=4
  Cos : Trigonometry  Operator=cos
  Gain : Gain  Gain=rc
  MATLAB Function1 : MATLAB Function  TreatAsAtomicUnit=on
  MATLAB Function4 : MATLAB Function  TreatAsAtomicUnit=on
  Product : Product
  Saturation : Saturate  UpperLimit=1  LowerLimit=-1
  Saturation1 : Saturate  UpperLimit=1  LowerLimit=-1
  Scope{,1..3} (4 alike) : Scope
  Sum : Sum  Inputs=|+-
  Switch : Switch
  Sigma5 : Outport
  alpha5 : Outport  Port=2
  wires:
  Thetad_5/1 -> Gain/1
  gamma5/1 -> Sum/1
  Gain/1 -> MATLAB Function4/1(v_wheel), MATLAB Function1/1(v_wheel)  "V_wheel"
  Switch/1 -> Scope/1, Sigma5/1
  MATLAB Function1/1(Fc_pos_out) -> Saturation/1
  MATLAB Function4/1(Fc_neg_out) -> Saturation1/1, Scope3/1
  Delta5/1 -> Sum/2
  Saturation/1 -> Scope2/1, Switch/1, Switch/2
  Saturation1/1 -> Switch/3
  Cos/1 -> Product/2
  Sum/1 -> Cos/1, Scope1/1, alpha5/1  "alpha1"
  Product/1 -> MATLAB Function1/2(Vx_DL), MATLAB Function4/2(Vx_DL)
  vx_ruota5/1 -> Product/1  "vx_ruota5"

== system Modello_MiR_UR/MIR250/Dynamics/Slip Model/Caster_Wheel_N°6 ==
  Thetad_6 : Inport
  vx_ruota6 : Inport  Port=2
  gamma6 : Inport  Port=3
  Delta6 : Inport  Port=4
  Cos : Trigonometry  Operator=cos
  Gain : Gain  Gain=rc
  MATLAB Function1 : MATLAB Function  TreatAsAtomicUnit=on
  MATLAB Function4 : MATLAB Function  TreatAsAtomicUnit=on
  Product : Product
  Saturation : Saturate  UpperLimit=1  LowerLimit=-1
  Saturation1 : Saturate  UpperLimit=1  LowerLimit=-1
  Scope{,1..3} (4 alike) : Scope
  Sum : Sum  Inputs=|+-
  Switch : Switch
  Sigma6 : Outport
  alpha6 : Outport  Port=2
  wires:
  Thetad_6/1 -> Gain/1
  gamma6/1 -> Sum/1
  Gain/1 -> MATLAB Function4/1(v_wheel), MATLAB Function1/1(v_wheel)  "V_wheel"
  Switch/1 -> Scope/1, Sigma6/1
  MATLAB Function1/1(Fc_pos_out) -> Saturation/1
  MATLAB Function4/1(Fc_neg_out) -> Saturation1/1, Scope3/1
  Delta6/1 -> Sum/2
  Saturation/1 -> Scope2/1, Switch/1, Switch/2
  Saturation1/1 -> Switch/3
  Cos/1 -> Product/2
  Sum/1 -> Cos/1, Scope1/1, alpha6/1  "alpha1"
  Product/1 -> MATLAB Function1/2(Vx_DL), MATLAB Function4/2(Vx_DL)
  vx_ruota6/1 -> Product/1  "xd_ruota6"

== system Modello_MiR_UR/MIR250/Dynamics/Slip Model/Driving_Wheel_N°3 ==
  Thetad_3 : Inport
  vx_ruota3 : Inport  Port=2
  gamma3 : Inport  Port=3
  Gain : Gain  Gain=rd
  MATLAB Function1 : MATLAB Function  TreatAsAtomicUnit=on
  MATLAB Function4 : MATLAB Function  TreatAsAtomicUnit=on
  Mux : Mux  Inputs=2
  Saturation : Saturate  UpperLimit=1  LowerLimit=-1
  Saturation1 : Saturate  UpperLimit=1  LowerLimit=-1
  Scope{,1..5} (6 alike) : Scope
  Switch : Switch
  Sigma3 : Outport
  alpha3 : Outport  Port=2
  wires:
  Thetad_3/1 -> Gain/1
  Gain/1 -> Mux/1, MATLAB Function4/1(v_wheel), MATLAB Function1/1(v_wheel)  "V_wheel"
  Switch/1 -> Scope/1, Sigma3/1
  MATLAB Function1/1(Fc_pos_out) -> Saturation1/1
  MATLAB Function4/1(Fc_neg_out) -> Saturation/1, Scope3/1
  vx_ruota3/1 -> MATLAB Function1/2(Vx_DL), MATLAB Function4/2(Vx_DL), Mux/2  "xd_ruota3"
  Saturation1/1 -> Scope2/1, Switch/1, Switch/2
  Saturation/1 -> Switch/3
  gamma3/1 -> Scope1/1, alpha3/1, Scope4/1
  Mux/1 -> Scope5/1

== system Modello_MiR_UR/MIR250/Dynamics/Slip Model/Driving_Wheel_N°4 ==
  Thetad_4 : Inport
  vx_ruota4 : Inport  Port=2
  gamma4 : Inport  Port=3
  Gain : Gain  Gain=rd
  MATLAB Function1 : MATLAB Function  TreatAsAtomicUnit=on
  MATLAB Function4 : MATLAB Function  TreatAsAtomicUnit=on
  Saturation : Saturate  UpperLimit=1  LowerLimit=-1
  Saturation1 : Saturate  UpperLimit=1  LowerLimit=-1
  Scope{,1..4} (5 alike) : Scope
  Switch : Switch
  Sigma4 : Outport
  alpha4 : Outport  Port=2
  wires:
  Thetad_4/1 -> Gain/1
  Gain/1 -> MATLAB Function4/1(v_wheel), MATLAB Function1/1(v_wheel)  "V_wheel"
  Switch/1 -> Scope/1, Sigma4/1
  MATLAB Function1/1(Fc_pos_out) -> Saturation1/1
  MATLAB Function4/1(Fc_neg_out) -> Saturation/1
  vx_ruota4/1 -> MATLAB Function4/2(Vx_DL), MATLAB Function1/2(Vx_DL)  "xd_ruota4"
  Saturation1/1 -> Scope2/1, Switch/1, Switch/2
  Saturation/1 -> Switch/3, Scope3/1
  gamma4/1 -> Scope1/1, alpha4/1, Scope4/1

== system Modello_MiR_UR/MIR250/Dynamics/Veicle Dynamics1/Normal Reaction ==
  Delta1 : Inport
  Delta2 : Inport  Port=2
  Delta5 : Inport  Port=3
  Delta6 : Inport  Port=4
  a_tau : Inport  Port=5
  a_n : Inport  Port=6
  Interpreted MATLAB Function : MATLABFcn  MATLABFcn=F63MIR(u)
  Interpreted MATLAB Function1 : MATLABFcn  MATLABFcn=F23MIR(u)
  Interpreted MATLAB Function2 : MATLABFcn  MATLABFcn=F43MIR(u)
  Interpreted MATLAB Function3 : MATLABFcn  MATLABFcn=mv*9.801-2*F63MIR(u)-2*F23MIR(u)-F43MIR(u)
  Mux9 : Mux  Inputs=6
  Saturation{,1..3} (4 alike) : Saturate  UpperLimit=inf  LowerLimit=0
  F13 : Outport  PortDimensions=1
  F23 : Outport  Port=2  PortDimensions=1
  F33 : Outport  Port=3  PortDimensions=1
  F43 : Outport  Port=4  PortDimensions=1
  F53 : Outport  Port=5  PortDimensions=1
  F63 : Outport  Port=6  PortDimensions=1
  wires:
  Delta1/1 -> Mux9/1
  a_n/1 -> Mux9/6
  Delta6/1 -> Mux9/4
  Interpreted MATLAB Function3/1 -> Saturation3/1
  Mux9/1 -> Interpreted MATLAB Function3/1, Interpreted MATLAB Function2/1, Interpreted MATLAB Function1/1, Interpreted MATLAB Function/1
  Delta5/1 -> Mux9/3
  a_tau/1 -> Mux9/5
  Interpreted MATLAB Function1/1 -> Saturation1/1  "F23"
  Delta2/1 -> Mux9/2
  Interpreted MATLAB Function/1 -> Saturation/1  "F63"
  Interpreted MATLAB Function2/1 -> Saturation2/1
  Saturation/1 -> F63/1, F53/1
  Saturation1/1 -> F23/1, F13/1
  Saturation2/1 -> F43/1
  Saturation3/1 -> F33/1

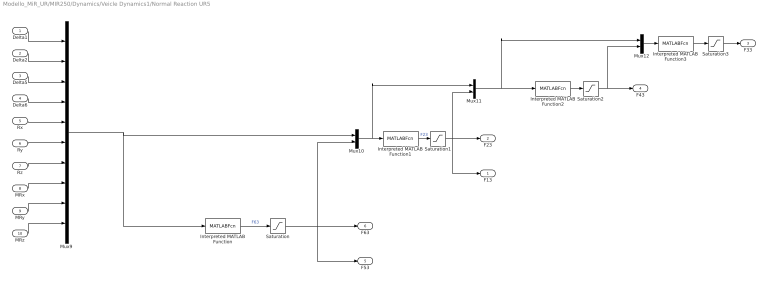
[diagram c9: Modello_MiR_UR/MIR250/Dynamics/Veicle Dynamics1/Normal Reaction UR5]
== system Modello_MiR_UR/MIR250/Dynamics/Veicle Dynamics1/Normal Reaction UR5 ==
  Delta1 : Inport
  Delta2 : Inport  Port=2
  Delta5 : Inport  Port=3
  Delta6 : Inport  Port=4
  Rx : Inport  Port=5
  Ry : Inport  Port=6
  Rz : Inport  Port=7
  MRx : Inport  Port=8
  MRy : Inport  Port=9
  MRz : Inport  Port=10
  Interpreted MATLAB Function : MATLABFcn  MATLABFcn=F63UR5(u)
  Interpreted MATLAB Function1 : MATLABFcn  MATLABFcn=F23UR5(u)
  Interpreted MATLAB Function2 : MATLABFcn  MATLABFcn=F43UR5(u)
  Interpreted MATLAB Function3 : MATLABFcn  MATLABFcn=2*u(12)+2*u(11)-u(13)
  Mux10 : Mux  Inputs=2
  Mux11 : Mux  Inputs=2
  Mux12 : Mux  Inputs=2
  Mux9 : Mux  Inputs=10
  Saturation{,1..3} (4 alike) : Saturate  UpperLimit=inf  LowerLimit=0
  F13 : Outport  PortDimensions=1
  F23 : Outport  Port=2  PortDimensions=1
  F33 : Outport  Port=3  PortDimensions=1
  F43 : Outport  Port=4  PortDimensions=1
  F53 : Outport  Port=5  PortDimensions=1
  F63 : Outport  Port=6  PortDimensions=1
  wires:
  Delta1/1 -> Mux9/1
  Mux10/1 -> Mux11/1, Interpreted MATLAB Function1/1
  Mux11/1 -> Interpreted MATLAB Function2/1, Mux12/1
  Delta6/1 -> Mux9/4
  Mux9/1 -> Mux10/1, Interpreted MATLAB Function/1
  Interpreted MATLAB Function3/1 -> Saturation3/1
  Mux12/1 -> Interpreted MATLAB Function3/1
  Delta5/1 -> Mux9/3
  Interpreted MATLAB Function1/1 -> Saturation1/1  "F23"
  Delta2/1 -> Mux9/2
  Interpreted MATLAB Function/1 -> Saturation/1  "F63"
  Interpreted MATLAB Function2/1 -> Saturation2/1
  Rx/1 -> Mux9/5
  Ry/1 -> Mux9/6
  Rz/1 -> Mux9/7
  MRx/1 -> Mux9/8
  MRy/1 -> Mux9/9
  MRz/1 -> Mux9/10
  Saturation/1 -> F63/1, F53/1, Mux10/2
  Saturation1/1 -> F23/1, F13/1, Mux11/2
  Saturation2/1 -> F43/1, Mux12/2
  Saturation3/1 -> F33/1

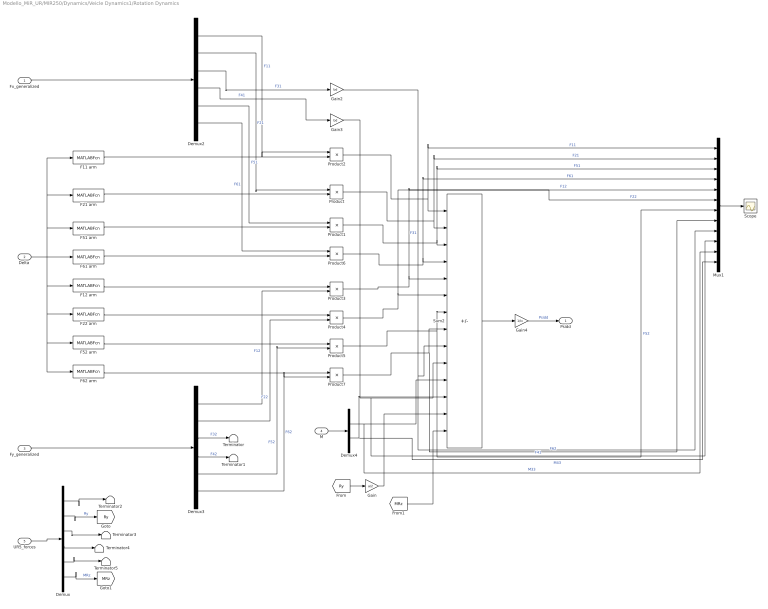
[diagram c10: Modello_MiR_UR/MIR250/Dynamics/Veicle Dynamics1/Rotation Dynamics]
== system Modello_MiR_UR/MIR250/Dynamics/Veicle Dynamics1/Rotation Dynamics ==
  Fx_generalized : Inport
  "Delta " : Inport  Port=2
  Fy_generalized : Inport  Port=3
  M : Inport  Port=4
  UR5_forces : Inport  Port=5
  Demux : Demux  Outputs=6
  Demux2 : Demux  Outputs=6
  Demux3 : Demux  Outputs=6
  Demux4 : Demux  Outputs=2
  F11 arm : MATLABFcn  MATLABFcn=b-b_caster*sin(u(1))
  F12 arm : MATLABFcn  MATLABFcn=a-b_caster*cos(u(1))
  F21 arm : MATLABFcn  MATLABFcn=b+b_caster*sin(u(2))
  F22 arm : MATLABFcn  MATLABFcn=a-b_caster*cos(u(2))
  F51 arm : MATLABFcn  MATLABFcn=b-b_caster*sin(u(3))
  F52 arm : MATLABFcn  MATLABFcn=a+b_caster*cos(u(3))
  F61 arm : MATLABFcn  MATLABFcn=b+b_caster*sin(u(4))
  F62 arm : MATLABFcn  MATLABFcn=a+b_caster*cos(u(4))
  Gain : Gain  Gain=a/2
  Gain2 : Gain  Gain=bd
  Gain3 : Gain  Gain=bd
  Gain4 : Gain  Gain=1/Iv
  Mux1 : Mux  Inputs=12
  Product{,1..7} (8 alike) : Product
  Scope : Scope
  Sum2 : Sum  Inputs=-+-+++---+++++
  Terminator{,1..5} (6 alike) : Terminator
  Psidd : Outport
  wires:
  Product2/1 -> Mux1/1, Sum2/1  "F11"
  Demux3/2 -> Product4/2  "F22"
  Sum2/1 -> Gain4/1
  Demux3/3 -> Terminator/1  "F32"
  Product4/1 -> Mux1/6, Sum2/6  "F22"
  Fx_generalized/1 -> Demux2/1
  Demux3/6 -> Product7/2  "F62"
  Demux2/2 -> Product/1  "F21"
  "Delta "/1 -> F51 arm/1, F21 arm/1, F11 arm/1, F62 arm/1, F52 arm/1, F22 arm/1, F12 arm/1, F61 arm/1
  Gain3/1 -> Sum2/10, Mux1/10  "F41"
  Product7/1 -> Mux1/8, Sum2/8  "F62"
  Gain2/1 -> Sum2/9, Mux1/9  "F31"
  Product3/1 -> Mux1/5, Sum2/5  "F12"
  Demux4/1 -> Sum2/11, Mux1/11  "M33"
  Demux3/4 -> Terminator1/1  "F42"
  Demux4/2 -> Mux1/12, Sum2/12  "M43"
  Demux2/1 -> Product2/1  "F11"
  Product/1 -> Mux1/2, Sum2/2  "F21"
  Gain4/1 -> Psidd/1  "Psidd"
  Demux2/3 -> Gain2/1  "F31"
  Demux2/4 -> Gain3/1  "F41"
  F51 arm/1 -> Product1/2
  Demux3/5 -> Product5/2  "F52"
  F61 arm/1 -> Product6/2
  Demux2/5 -> Product1/1  "F51"
  Product5/1 -> Mux1/7, Sum2/7  "F52"
  F21 arm/1 -> Product/2
  Demux3/1 -> Product3/2  "F12"
  Product1/1 -> Mux1/3, Sum2/3  "F51"
  Demux2/6 -> Product6/1  "F61"
  F11 arm/1 -> Product2/2
  Product6/1 -> Mux1/4, Sum2/4  "F61"
  Fy_generalized/1 -> Demux3/1
  Mux1/1 -> Scope/1
  F22 arm/1 -> Product4/1
  F52 arm/1 -> Product5/1
  F62 arm/1 -> Product7/1
  F12 arm/1 -> Product3/1
  M/1 -> Demux4/1
  UR5_forces/1 -> Demux/1
  Demux/2 -> [Ry]  "Ry"
  [Ry] -> Gain/1
  Gain/1 -> Sum2/13
  Demux/6 -> [MRz]  "MRz"
  [MRz] -> Sum2/14
  Demux/1 -> Terminator2/1
  Demux/3 -> Terminator3/1
  Demux/4 -> Terminator4/1
  Demux/5 -> Terminator5/1

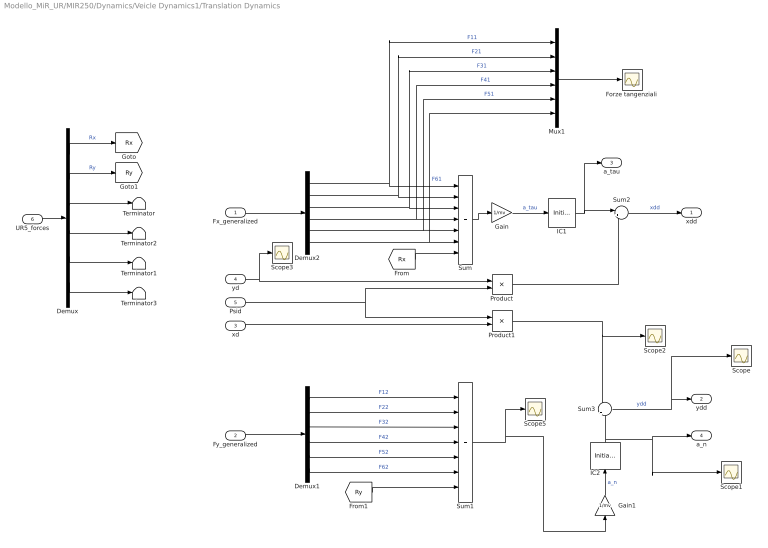
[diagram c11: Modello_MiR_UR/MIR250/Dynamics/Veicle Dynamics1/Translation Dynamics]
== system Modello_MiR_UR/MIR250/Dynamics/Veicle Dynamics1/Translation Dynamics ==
  Fx_generalized : Inport
  Fy_generalized : Inport  Port=2
  xd : Inport  Port=3
  yd : Inport  Port=4
  Psid : Inport  Port=5
  UR5_forces : Inport  Port=6
  Demux : Demux  Outputs=6
  Demux1 : Demux  Outputs=6
  Demux2 : Demux  Outputs=6
  Forze tangenziali : Scope
  Gain : Gain  Gain=1/mv
  Gain1 : Gain  Gain=1/mv
  IC1 : InitialCondition  Value=0
  IC2 : InitialCondition  Value=0
  Mux1 : Mux  Inputs=6
  Product : Product
  Product1 : Product
  Scope{,1..3,5} (5 alike) : Scope
  Sum : Sum  Inputs=7
  Sum1 : Sum  Inputs=7
  Sum2 : Sum  Inputs=|++
  Sum3 : Sum  Inputs=-|+
  Terminator{,1..3} (4 alike) : Terminator
  xdd : Outport
  ydd : Outport  Port=2
  a_tau : Outport  Port=3  PortDimensions=1
  a_n : Outport  Port=4  PortDimensions=1
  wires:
  Demux1/1 -> Sum1/1  "F12"
  Demux1/2 -> Sum1/2  "F22"
  Sum3/1 -> Scope/1, ydd/1  "ydd"
  Demux1/3 -> Sum1/3  "F32"
  Demux2/4 -> Mux1/4, Sum/4  "F41"
  Demux2/5 -> Mux1/5, Sum/5  "F51"
  Fx_generalized/1 -> Demux2/1
  Demux2/2 -> Sum/2, Mux1/2  "F21"
  Demux1/4 -> Sum1/4  "F42"
  Demux2/3 -> Mux1/3, Sum/3  "F31"
  Demux2/1 -> Sum/1, Mux1/1  "F11"
  Demux1/5 -> Sum1/5  "F52"
  Demux2/6 -> Mux1/6, Sum/6  "F61"
  Demux1/6 -> Sum1/6  "F62"
  Fy_generalized/1 -> Demux1/1
  Sum/1 -> Gain/1
  yd/1 -> Scope3/1, Product/1
  Psid/1 -> Product1/1, Product/2
  Gain/1 -> IC1/1  "a_tau"
  Product/1 -> Sum2/2
  xd/1 -> Product1/2
  Gain1/1 -> IC2/1  "a_n"
  Product1/1 -> Scope2/1, Sum3/1
  Mux1/1 -> Forze tangenziali/1
  IC1/1 -> Sum2/1, a_tau/1
  Sum2/1 -> xdd/1  "xdd"
  IC2/1 -> Sum3/2, Scope1/1, a_n/1
  Sum1/1 -> Gain1/1, Scope5/1
  UR5_forces/1 -> Demux/1
  Demux/1 -> [Rx]  "Rx"
  [Rx] -> Sum/7
  Demux/2 -> [Ry]  "Ry"
  [Ry] -> Sum1/7
  Demux/3 -> Terminator/1
  Demux/4 -> Terminator2/1
  Demux/5 -> Terminator1/1
  Demux/6 -> Terminator3/1
